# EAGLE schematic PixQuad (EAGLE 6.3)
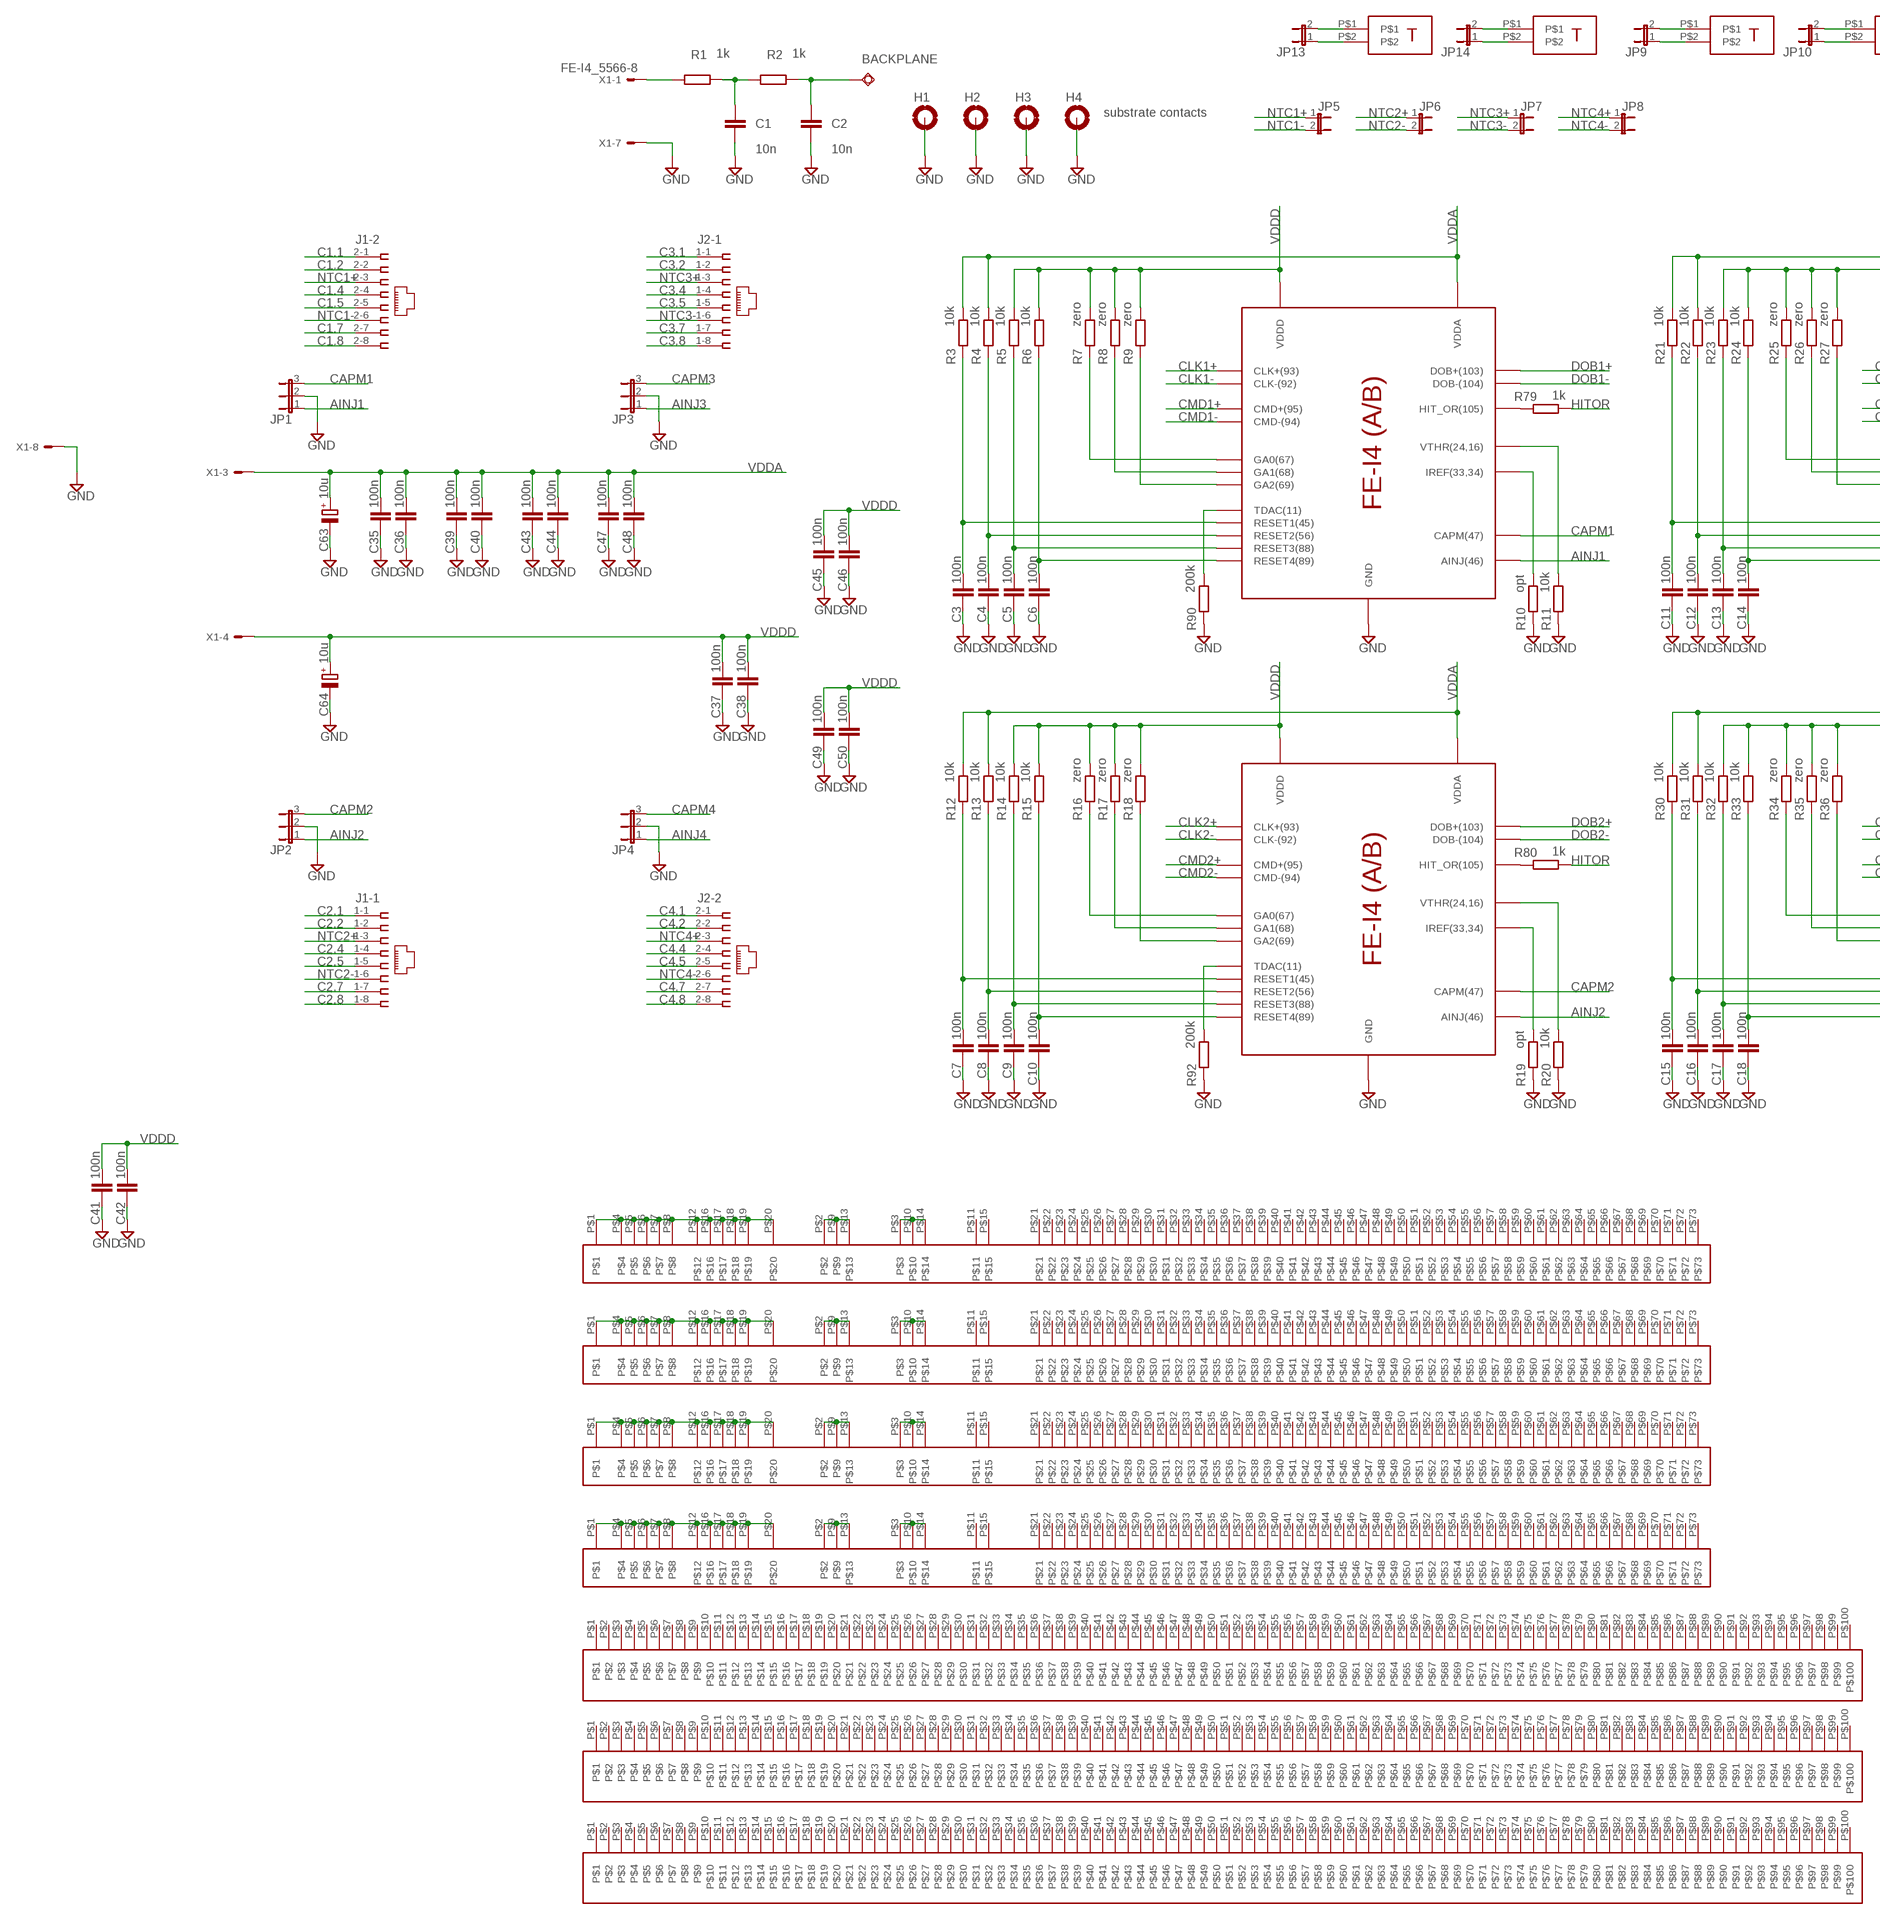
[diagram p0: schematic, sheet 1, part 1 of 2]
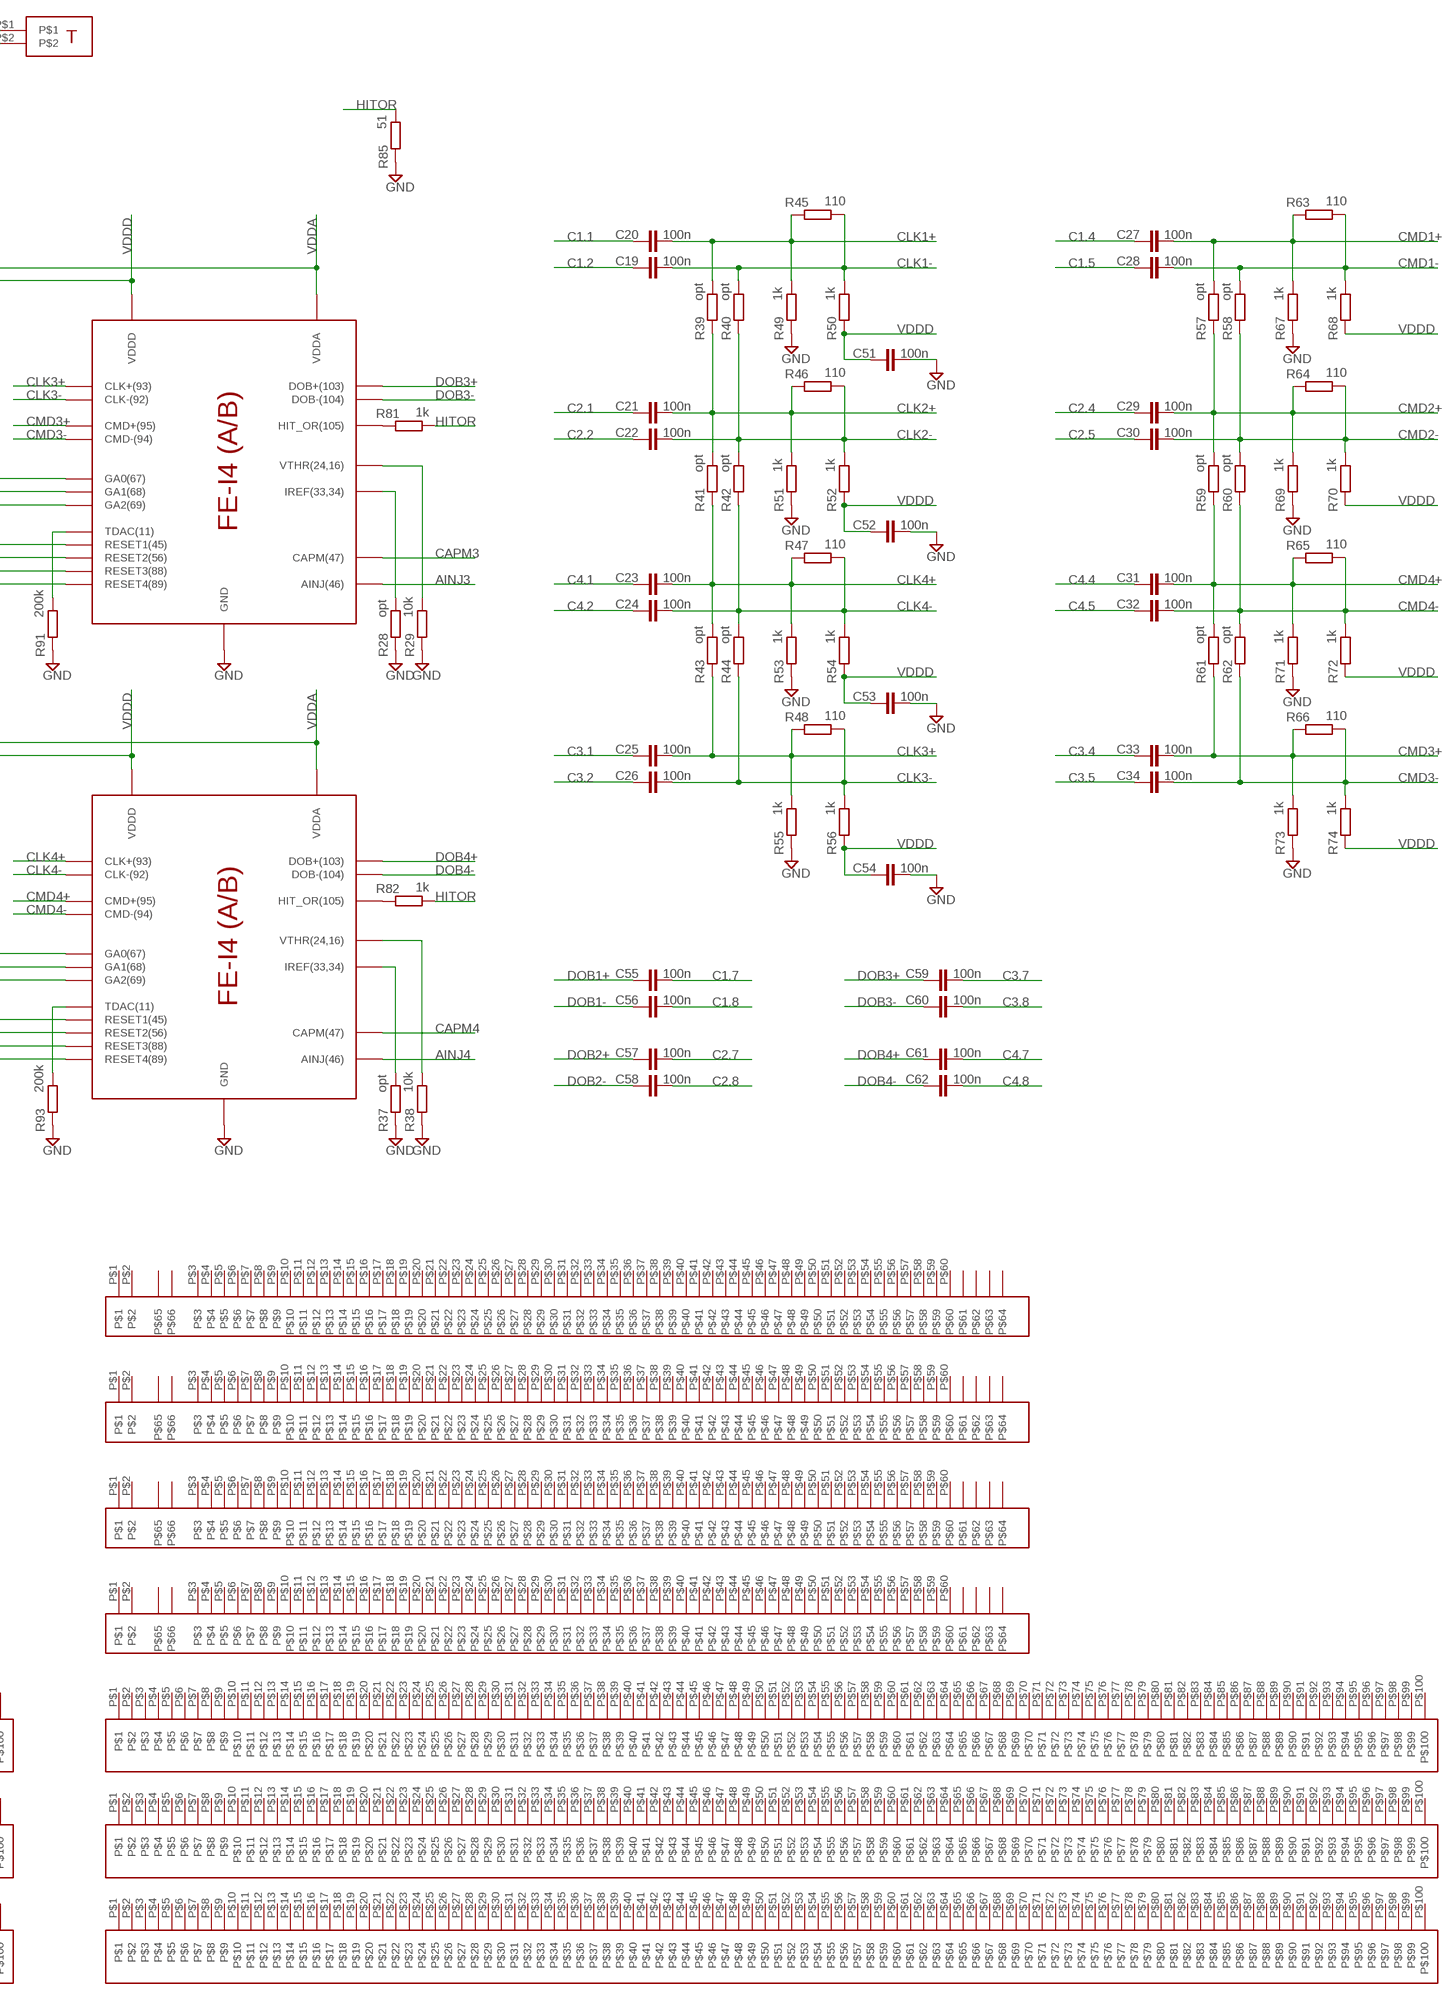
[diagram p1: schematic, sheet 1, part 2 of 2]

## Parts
BACKPLANE  TPSQTP20SQ  [TP20SQ]
C1  10n  C-EUC1210  [C1210]
C2  10n  C-EUC1210  [C1210]
C3  100n  C-EUC0402  [C0402]
C4  100n  C-EUC0402  [C0402]
C5  100n  C-EUC0402  [C0402]
C6  100n  C-EUC0402  [C0402]
C7  100n  C-EUC0402  [C0402]
C8  100n  C-EUC0402  [C0402]
C9  100n  C-EUC0402  [C0402]
C10  100n  C-EUC0402  [C0402]
C11  100n  C-EUC0402  [C0402]
C12  100n  C-EUC0402  [C0402]
C13  100n  C-EUC0402  [C0402]
C14  100n  C-EUC0402  [C0402]
C15  100n  C-EUC0402  [C0402]
C16  100n  C-EUC0402  [C0402]
C17  100n  C-EUC0402  [C0402]
C18  100n  C-EUC0402  [C0402]
C19  100n  C-EUC0402  [C0402]
C20  100n  C-EUC0402  [C0402]
C21  100n  C-EUC0402  [C0402]
C22  100n  C-EUC0402  [C0402]
C23  100n  C-EUC0402  [C0402]
C24  100n  C-EUC0402  [C0402]
C25  100n  C-EUC0402  [C0402]
C26  100n  C-EUC0402  [C0402]
C27  100n  C-EUC0402  [C0402]
C28  100n  C-EUC0402  [C0402]
C29  100n  C-EUC0402  [C0402]
C30  100n  C-EUC0402  [C0402]
C31  100n  C-EUC0402  [C0402]
C32  100n  C-EUC0402  [C0402]
C33  100n  C-EUC0402  [C0402]
C34  100n  C-EUC0402  [C0402]
C35  100n  C-EUC0402  [C0402]
C36  100n  C-EUC0402  [C0402]
C37  100n  C-EUC0402  [C0402]
C38  100n  C-EUC0402  [C0402]
C39  100n  C-EUC0402  [C0402]
C40  100n  C-EUC0402  [C0402]
C41  100n  C-EUC0402  [C0402]
C42  100n  C-EUC0402  [C0402]
C43  100n  C-EUC0402  [C0402]
C44  100n  C-EUC0402  [C0402]
C45  100n  C-EUC0402  [C0402]
C46  100n  C-EUC0402  [C0402]
C47  100n  C-EUC0402  [C0402]
C48  100n  C-EUC0402  [C0402]
C49  100n  C-EUC0402  [C0402]
C50  100n  C-EUC0402  [C0402]
C51  100n  C-EUC0402  [C0402]
C52  100n  C-EUC0402  [C0402]
C53  100n  C-EUC0402  [C0402]
C54  100n  C-EUC0402  [C0402]
C55  100n  C-EUC0402  [C0402]
C56  100n  C-EUC0402  [C0402]
C57  100n  C-EUC0402  [C0402]
C58  100n  C-EUC0402  [C0402]
C59  100n  C-EUC0402  [C0402]
C60  100n  C-EUC0402  [C0402]
C61  100n  C-EUC0402  [C0402]
C62  100n  C-EUC0402  [C0402]
C63  10u  CPOL-EUCT3528  [CT3528]
C64  10u  CPOL-EUCT3528  [CT3528]
H1  MOUNT-PAD-ROUND3.2  [3,2-PAD]
H2  MOUNT-PAD-ROUND3.2  [3,2-PAD]
H3  MOUNT-PAD-ROUND3.2  [3,2-PAD]
H4  substrate contacts  MOUNT-PAD-ROUND3.2  [3,2-PAD]
J1  557560-1  [557560-1]
J2  557560-1  [557560-1]
JP1  JP2E  [JP2]
JP2  JP2E  [JP2]
JP3  JP2E  [JP2]
JP4  JP2E  [JP2]
JP5  JP1E  [JP1]
JP6  JP1E  [JP1]
JP7  JP1E  [JP1]
JP8  JP1E  [JP1]
JP9  JP1E  [JUMPER_JP1]
JP10  JP1E  [JUMPER_JP1]
JP13  JP1E  [JUMPER_JP1]
JP14  JP1E  [JUMPER_JP1]
R1  1k  R-EU_R1206  [R1206]
R2  1k  R-EU_R1206  [R1206]
R3  10k  R-EU_R0402  [R0402]
R4  10k  R-EU_R0402  [R0402]
R5  10k  R-EU_R0402  [R0402]
R6  10k  R-EU_R0402  [R0402]
R7  zero  R-EU_R0402  [R0402]
R8  zero  R-EU_R0402  [R0402]
R9  zero  R-EU_R0402  [R0402]
R10  opt  R-EU_R0402  [R0402]
R11  10k  R-EU_R0402  [R0402]
R12  10k  R-EU_R0402  [R0402]
R13  10k  R-EU_R0402  [R0402]
R14  10k  R-EU_R0402  [R0402]
R15  10k  R-EU_R0402  [R0402]
R16  zero  R-EU_R0402  [R0402]
R17  zero  R-EU_R0402  [R0402]
R18  zero  R-EU_R0402  [R0402]
R19  opt  R-EU_R0402  [R0402]
R20  10k  R-EU_R0402  [R0402]
R21  10k  R-EU_R0402  [R0402]
R22  10k  R-EU_R0402  [R0402]
R23  10k  R-EU_R0402  [R0402]
R24  10k  R-EU_R0402  [R0402]
R25  zero  R-EU_R0402  [R0402]
R26  zero  R-EU_R0402  [R0402]
R27  zero  R-EU_R0402  [R0402]
R28  opt  R-EU_R0402  [R0402]
R29  10k  R-EU_R0402  [R0402]
R30  10k  R-EU_R0402  [R0402]
R31  10k  R-EU_R0402  [R0402]
R32  10k  R-EU_R0402  [R0402]
R33  10k  R-EU_R0402  [R0402]
R34  zero  R-EU_R0402  [R0402]
R35  zero  R-EU_R0402  [R0402]
R36  zero  R-EU_R0402  [R0402]
R37  opt  R-EU_R0402  [R0402]
R38  10k  R-EU_R0402  [R0402]
R39  opt  R-EU_R0402  [R0402]
R40  opt  R-EU_R0402  [R0402]
R41  opt  R-EU_R0402  [R0402]
R42  opt  R-EU_R0402  [R0402]
R43  opt  R-EU_R0402  [R0402]
R44  opt  R-EU_R0402  [R0402]
R45  110  R-EU_R0402  [R0402]
R46  110  R-EU_R0402  [R0402]
R47  110  R-EU_R0402  [R0402]
R48  110  R-EU_R0402  [R0402]
R49  1k  R-EU_R0402  [R0402]
R50  1k  R-EU_R0402  [R0402]
R51  1k  R-EU_R0402  [R0402]
R52  1k  R-EU_R0402  [R0402]
R53  1k  R-EU_R0402  [R0402]
R54  1k  R-EU_R0402  [R0402]
R55  1k  R-EU_R0402  [R0402]
R56  1k  R-EU_R0402  [R0402]
R57  opt  R-EU_R0402  [R0402]
R58  opt  R-EU_R0402  [R0402]
R59  opt  R-EU_R0402  [R0402]
R60  opt  R-EU_R0402  [R0402]
R61  opt  R-EU_R0402  [R0402]
R62  opt  R-EU_R0402  [R0402]
R63  110  R-EU_R0402  [R0402]
R64  110  R-EU_R0402  [R0402]
R65  110  R-EU_R0402  [R0402]
R66  110  R-EU_R0402  [R0402]
R67  1k  R-EU_R0402  [R0402]
R68  1k  R-EU_R0402  [R0402]
R69  1k  R-EU_R0402  [R0402]
R70  1k  R-EU_R0402  [R0402]
R71  1k  R-EU_R0402  [R0402]
R72  1k  R-EU_R0402  [R0402]
R73  1k  R-EU_R0402  [R0402]
R74  1k  R-EU_R0402  [R0402]
R79  1k  R-EU_R0402  [R0402]
R80  1k  R-EU_R0402  [R0402]
R81  1k  R-EU_R0402  [R0402]
R82  1k  R-EU_R0402  [R0402]
R85  51  RCL_R-EU_R0603  [RCL_R0603]
R90  200k  R-EU_R0402  [R0402]
R91  200k  R-EU_R0402  [R0402]
R92  200k  R-EU_R0402  [R0402]
R93  200k  R-EU_R0402  [R0402]
U$1  FE_I4ASIC  [FE-I4]
U$2  FE_I4ASIC  [FE-I4]
U$3  FE_I4ASIC  [FE-I4]
U$4  FE_I4ASIC  [FE-I4]
U$5  PA2  [PA2]
U$6  PA2  [PA2]
U$7  PA2  [PA2]
U$8  PA2  [PA2]
U$9  PA2  [PA2]
U$10  PA2  [PA2]
U$11  PA3  [PA3]
U$12  PA1  [PA1]
U$13  PA1  [PA1]
U$14  PA1  [PA1]
U$15  PA1  [PA1]
U$16  PA3  [PA3]
U$17  DORT  [DORT]
U$18  DORT  [DORT]
U$19  PA3  [PA3]
U$20  PA3  [PA3]
U$21  DORT  [DORT]
U$22  DORT  [DORT]
X1  FE-I4_5566-8  [FE-I4_5566-8]

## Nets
AINJ1: JP1.1 U$1.AINJ(46)
AINJ2: JP2.1 U$2.AINJ(46)
AINJ3: JP3.1 U$3.AINJ(46)
AINJ4: JP4.1 U$4.AINJ(46)
C1.1: C20.2 J1.2-1
C1.2: C19.2 J1.2-2
C1.4: C27.2 J1.2-4
C1.5: C28.2 J1.2-5
C1.7: C55.1 J1.2-7
C1.8: C56.1 J1.2-8
C2.1: C21.2 J1.1-1
C2.2: C22.2 J1.1-2
C2.4: C29.2 J1.1-4
C2.5: C30.2 J1.1-5
C2.7: C57.1 J1.1-7
C2.8: C58.1 J1.1-8
C3.1: C25.2 J2.1-1
C3.2: C26.2 J2.1-2
C3.4: C33.2 J2.1-4
C3.5: C34.2 J2.1-5
C3.7: C59.1 J2.1-7
C3.8: C60.1 J2.1-8
C4.1: C23.2 J2.2-1
C4.2: C24.2 J2.2-2
C4.4: C31.2 J2.2-4
C4.5: C32.2 J2.2-5
C4.7: C61.1 J2.2-7
C4.8: C62.1 J2.2-8
CAPM1: JP1.3 U$1.CAPM(47)
CAPM2: JP2.3 U$2.CAPM(47)
CAPM3: JP3.3 U$3.CAPM(47)
CAPM4: JP4.3 U$4.CAPM(47)
CLK1+: C20.1 R39.2 R45.1 R49.2 U$1.CLK+(93)
CLK1-: C19.1 R40.2 R45.2 R50.2 U$1.CLK-(92)
CLK2+: C21.1 R39.1 R41.2 R46.1 R51.2 U$2.CLK+(93)
CLK2-: C22.1 R40.1 R42.2 R46.2 R52.2 U$2.CLK-(92)
CLK3+: C25.1 R43.1 R48.1 R55.2 U$3.CLK+(93)
CLK3-: C26.1 R44.1 R48.2 R56.2 U$3.CLK-(92)
CLK4+: C23.1 R41.1 R43.2 R47.1 R53.2 U$4.CLK+(93)
CLK4-: C24.1 R42.1 R44.2 R47.2 R54.2 U$4.CLK-(92)
CMD1+: C27.1 R57.2 R63.1 R67.2 U$1.CMD+(95)
CMD1-: C28.1 R58.2 R63.2 R68.2 U$1.CMD-(94)
CMD2+: C29.1 R57.1 R59.2 R64.1 R69.2 U$2.CMD+(95)
CMD2-: C30.1 R58.1 R60.2 R64.2 R70.2 U$2.CMD-(94)
CMD3+: C33.1 R61.1 R66.1 R73.2 U$3.CMD+(95)
CMD3-: C34.1 R62.1 R66.2 R74.2 U$3.CMD-(94)
CMD4+: C31.1 R59.1 R61.2 R65.1 R71.2 U$4.CMD+(95)
CMD4-: C32.1 R60.1 R62.2 R65.2 R72.2 U$4.CMD-(94)
DOB1+: C55.2 U$1.DOB+(103)
DOB1-: C56.2 U$1.DOB-(104)
DOB2+: C57.2 U$2.DOB+(103)
DOB2-: C58.2 U$2.DOB-(104)
DOB3+: C59.2 U$3.DOB+(103)
DOB3-: C60.2 U$3.DOB-(104)
DOB4+: C61.2 U$4.DOB+(103)
DOB4-: C62.2 U$4.DOB-(104)
GND: C1.2 C2.2 C3.2 C4.2 C5.2 C6.2 C7.2 C8.2 C9.2 C10.2 C11.2 C12.2 C13.2 C14.2 C15.2 C16.2 C17.2 C18.2 C35.2 C36.2 C37.2 C38.2 C39.2 C40.2 C41.2 C42.2 C43.2 C44.2 C45.2 C46.2 C47.2 C48.2 C49.2 C50.2 C51.1 C52.1 C53.1 C54.1 C63.- C64.- H1.B3,2(MOUNT) H2.B3,2(MOUNT) H3.B3,2(MOUNT) H4.B3,2(MOUNT) JP1.2 JP2.2 JP3.2 JP4.2 R10.1 R11.1 R19.1 R20.1 R28.1 R29.1 R37.1 R38.1 R49.1 R51.1 R53.1 R55.1 R67.1 R69.1 R71.1 R73.1 R85.1 R90.1 R91.1 R92.1 R93.1 U$1.GND U$2.GND U$3.GND U$4.GND X1.7 X1.8
HITOR: R79.2 R80.2 R81.2 R82.2 R85.2
N$1: BACKPLANE.TP C2.1 R2.2
N$2: C1.1 R1.2 R2.1
N$3: JP13.2 U$17.P$1
N$4: C3.1 R3.1 U$1.RESET1(45)
N$5: C4.1 R4.1 U$1.RESET2(56)
N$6: C5.1 R5.1 U$1.RESET3(88)
N$7: C6.1 R6.1 U$1.RESET4(89)
N$8: R7.1 U$1.GA0(67)
N$9: R8.1 U$1.GA1(68)
N$10: R9.1 U$1.GA2(69)
N$11: R10.2 U$1.IREF(33,34)
N$12: R11.2 U$1.VTHR(24,16)
N$13: R79.1 U$1.P$1(HIT_OR(105))
N$14: R16.1 U$2.GA0(67)
N$15: R17.1 U$2.GA1(68)
N$16: R18.1 U$2.GA2(69)
N$17: C7.1 R12.1 U$2.RESET1(45)
N$18: C8.1 R13.1 U$2.RESET2(56)
N$19: C9.1 R14.1 U$2.RESET3(88)
N$20: C10.1 R15.1 U$2.RESET4(89)
N$21: R80.1 U$2.P$1(HIT_OR(105))
N$22: R81.1 U$3.P$1(HIT_OR(105))
N$23: R82.1 U$4.P$1(HIT_OR(105))
N$24: R90.2 U$1.TDAC(11)
N$25: R19.2 U$2.IREF(33,34)
N$26: R20.2 U$2.VTHR(24,16)
N$27: R91.2 U$3.TDAC(11)
N$28: R92.2 U$2.TDAC(11)
N$29: R93.2 U$4.TDAC(11)
N$30: JP13.1 U$17.P$2
N$31: JP14.1 U$18.P$2
N$32: JP14.2 U$18.P$1
N$33: U$11.P$1 U$11.P$4 U$11.P$5 U$11.P$6 U$11.P$7 U$11.P$8 U$11.P$12 U$11.P$16 U$11.P$17 U$11.P$18 U$11.P$19 U$11.P$20
N$34: R1.1 X1.1
N$35: U$16.P$1 U$16.P$4 U$16.P$5 U$16.P$6 U$16.P$7 U$16.P$8 U$16.P$12 U$16.P$16 U$16.P$17 U$16.P$18 U$16.P$19 U$16.P$20
N$36: U$19.P$1 U$19.P$4 U$19.P$5 U$19.P$6 U$19.P$7 U$19.P$8 U$19.P$12 U$19.P$16 U$19.P$17 U$19.P$18 U$19.P$19 U$19.P$20
N$37: U$20.P$1 U$20.P$4 U$20.P$5 U$20.P$6 U$20.P$7 U$20.P$8 U$20.P$12 U$20.P$16 U$20.P$17 U$20.P$18 U$20.P$19 U$20.P$20
N$38: U$11.P$2 U$11.P$9 U$11.P$13
N$39: U$16.P$2 U$16.P$9 U$16.P$13
N$40: U$19.P$2 U$19.P$9 U$19.P$13
N$41: U$20.P$2 U$20.P$9 U$20.P$13
N$42: U$20.P$3 U$20.P$10 U$20.P$14
N$43: U$19.P$3 U$19.P$10 U$19.P$14
N$44: U$16.P$3 U$16.P$10 U$16.P$14
N$45: U$11.P$3 U$11.P$10 U$11.P$14
N$46: JP9.1 U$21.P$2
N$47: JP9.2 U$21.P$1
N$48: JP10.1 U$22.P$2
N$49: JP10.2 U$22.P$1
N$50: R27.1 U$3.GA2(69)
N$56: R28.2 U$3.IREF(33,34)
N$57: R26.1 U$3.GA1(68)
N$58: R25.1 U$3.GA0(67)
N$59: C11.1 R21.1 U$3.RESET1(45)
N$60: C12.1 R22.1 U$3.RESET2(56)
N$61: C13.1 R23.1 U$3.RESET3(88)
N$62: C14.1 R24.1 U$3.RESET4(89)
N$64: R29.2 U$3.VTHR(24,16)
N$73: R34.1 U$4.GA0(67)
N$74: R35.1 U$4.GA1(68)
N$75: R36.1 U$4.GA2(69)
N$76: C15.1 R30.1 U$4.RESET1(45)
N$77: C16.1 R31.1 U$4.RESET2(56)
N$78: C17.1 R32.1 U$4.RESET3(88)
N$79: C18.1 R33.1 U$4.RESET4(89)
N$80: R37.2 U$4.IREF(33,34)
N$81: R38.2 U$4.VTHR(24,16)
NTC1+: J1.2-3 JP5.1
NTC1-: J1.2-6 JP5.2
NTC2+: J1.1-3 JP6.1
NTC2-: J1.1-6 JP6.2
NTC3+: J2.1-3 JP7.1
NTC3-: J2.1-6 JP7.2
NTC4+: J2.2-3 JP8.1
NTC4-: J2.2-6 JP8.2
VDDA: C35.1 C36.1 C39.1 C40.1 C43.1 C44.1 C47.1 C48.1 C63.+ R3.2 R4.2 R12.2 R13.2 R21.2 R22.2 R30.2 R31.2 U$1.VDDA U$2.VDDA U$3.VDDA U$4.VDDA X1.3
VDDD: C37.1 C38.1 C41.1 C42.1 C45.1 C46.1 C49.1 C50.1 C51.2 C52.2 C53.2 C54.2 C64.+ R5.2 R6.2 R7.2 R8.2 R9.2 R14.2 R15.2 R16.2 R17.2 R18.2 R23.2 R24.2 R25.2 R26.2 R27.2 R32.2 R33.2 R34.2 R35.2 R36.2 R50.1 R52.1 R54.1 R56.1 R68.1 R70.1 R72.1 R74.1 U$1.VDDD U$2.VDDD U$3.VDDD U$4.VDDD X1.4
Unconnected: U$5.P$1 U$5.P$2 U$5.P$3 U$5.P$4 U$5.P$5 U$5.P$6 U$5.P$7 U$5.P$8 U$5.P$9 U$5.P$10 U$5.P$11 U$5.P$12 U$5.P$13 U$5.P$14 U$5.P$15 U$5.P$16 U$5.P$17 U$5.P$18 U$5.P$19 U$5.P$20 U$5.P$21 U$5.P$22 U$5.P$23 U$5.P$24 U$5.P$25 U$5.P$26 U$5.P$27 U$5.P$28 U$5.P$29 U$5.P$30 U$5.P$31 U$5.P$32 U$5.P$33 U$5.P$34 U$5.P$35 U$5.P$36 U$5.P$37 U$5.P$38 U$5.P$39 U$5.P$40 U$5.P$41 U$5.P$42 U$5.P$43 U$5.P$44 U$5.P$45 U$5.P$46 U$5.P$47 U$5.P$48 U$5.P$49 U$5.P$50 U$5.P$51 U$5.P$52 U$5.P$53 U$5.P$54 U$5.P$55 U$5.P$56 U$5.P$57 U$5.P$58 U$5.P$59 U$5.P$60 U$5.P$61 U$5.P$62 U$5.P$63 U$5.P$64 U$5.P$65 U$5.P$66 U$5.P$67 U$5.P$68 U$5.P$69 U$5.P$70 U$5.P$71 U$5.P$72 U$5.P$73 U$5.P$74 U$5.P$75 U$5.P$76 U$5.P$77 U$5.P$78 U$5.P$79 U$5.P$80 U$5.P$81 U$5.P$82 U$5.P$83 U$5.P$84 U$5.P$85 U$5.P$86 U$5.P$87 U$5.P$88 U$5.P$89 U$5.P$90 U$5.P$91 U$5.P$92 U$5.P$93 U$5.P$94 U$5.P$95 U$5.P$96 U$5.P$97 U$5.P$98 U$5.P$99 U$5.P$100 U$6.P$1 U$6.P$2 U$6.P$3 U$6.P$4 U$6.P$5 U$6.P$6 U$6.P$7 U$6.P$8 U$6.P$9 U$6.P$10 U$6.P$11 U$6.P$12 U$6.P$13 U$6.P$14 U$6.P$15 U$6.P$16 U$6.P$17 U$6.P$18 U$6.P$19 U$6.P$20 U$6.P$21 U$6.P$22 U$6.P$23 U$6.P$24 U$6.P$25 U$6.P$26 U$6.P$27 U$6.P$28 U$6.P$29 U$6.P$30 U$6.P$31 U$6.P$32 U$6.P$33 U$6.P$34 U$6.P$35 U$6.P$36 U$6.P$37 U$6.P$38 U$6.P$39 U$6.P$40 U$6.P$41 U$6.P$42 U$6.P$43 U$6.P$44 U$6.P$45 U$6.P$46 U$6.P$47 U$6.P$48 U$6.P$49 U$6.P$50 U$6.P$51 U$6.P$52 U$6.P$53 U$6.P$54 U$6.P$55 U$6.P$56 U$6.P$57 U$6.P$58 U$6.P$59 U$6.P$60 U$6.P$61 U$6.P$62 U$6.P$63 U$6.P$64 U$6.P$65 U$6.P$66 U$6.P$67 U$6.P$68 U$6.P$69 U$6.P$70 U$6.P$71 U$6.P$72 U$6.P$73 U$6.P$74 U$6.P$75 U$6.P$76 U$6.P$77 U$6.P$78 U$6.P$79 U$6.P$80 U$6.P$81 U$6.P$82 U$6.P$83 U$6.P$84 U$6.P$85 U$6.P$86 U$6.P$87 U$6.P$88 U$6.P$89 U$6.P$90 U$6.P$91 U$6.P$92 U$6.P$93 U$6.P$94 U$6.P$95 U$6.P$96 U$6.P$97 U$6.P$98 U$6.P$99 U$6.P$100 U$7.P$1 U$7.P$2 U$7.P$3 U$7.P$4 U$7.P$5 U$7.P$6 U$7.P$7 U$7.P$8 U$7.P$9 U$7.P$10 U$7.P$11 U$7.P$12 U$7.P$13 U$7.P$14 U$7.P$15 U$7.P$16 U$7.P$17 U$7.P$18 U$7.P$19 U$7.P$20 U$7.P$21 U$7.P$22 U$7.P$23 U$7.P$24 U$7.P$25 U$7.P$26 U$7.P$27 U$7.P$28 U$7.P$29 U$7.P$30 U$7.P$31 U$7.P$32 U$7.P$33 U$7.P$34 U$7.P$35 U$7.P$36 U$7.P$37 U$7.P$38 U$7.P$39 U$7.P$40 U$7.P$41 U$7.P$42 U$7.P$43 U$7.P$44 U$7.P$45 U$7.P$46 U$7.P$47 U$7.P$48 U$7.P$49 U$7.P$50 U$7.P$51 U$7.P$52 U$7.P$53 U$7.P$54 U$7.P$55 U$7.P$56 U$7.P$57 U$7.P$58 U$7.P$59 U$7.P$60 U$7.P$61 U$7.P$62 U$7.P$63 U$7.P$64 U$7.P$65 U$7.P$66 U$7.P$67 U$7.P$68 U$7.P$69 U$7.P$70 U$7.P$71 U$7.P$72 U$7.P$73 U$7.P$74 U$7.P$75 U$7.P$76 U$7.P$77 U$7.P$78 U$7.P$79 U$7.P$80 U$7.P$81 U$7.P$82 U$7.P$83 U$7.P$84 U$7.P$85 U$7.P$86 U$7.P$87 U$7.P$88 U$7.P$89 U$7.P$90 U$7.P$91 U$7.P$92 U$7.P$93 U$7.P$94 U$7.P$95 U$7.P$96 U$7.P$97 U$7.P$98 U$7.P$99 U$7.P$100 U$8.P$1 U$8.P$2 U$8.P$3 U$8.P$4 U$8.P$5 U$8.P$6 U$8.P$7 U$8.P$8 U$8.P$9 U$8.P$10 U$8.P$11 U$8.P$12 U$8.P$13 U$8.P$14 U$8.P$15 U$8.P$16 U$8.P$17 U$8.P$18 U$8.P$19 U$8.P$20 U$8.P$21 U$8.P$22 U$8.P$23 U$8.P$24 U$8.P$25 U$8.P$26 U$8.P$27 U$8.P$28 U$8.P$29 U$8.P$30 U$8.P$31 U$8.P$32 U$8.P$33 U$8.P$34 U$8.P$35 U$8.P$36 U$8.P$37 U$8.P$38 U$8.P$39 U$8.P$40 U$8.P$41 U$8.P$42 U$8.P$43 U$8.P$44 U$8.P$45 U$8.P$46 U$8.P$47 U$8.P$48 U$8.P$49 U$8.P$50 U$8.P$51 U$8.P$52 U$8.P$53 U$8.P$54 U$8.P$55 U$8.P$56 U$8.P$57 U$8.P$58 U$8.P$59 U$8.P$60 U$8.P$61 U$8.P$62 U$8.P$63 U$8.P$64 U$8.P$65 U$8.P$66 U$8.P$67 U$8.P$68 U$8.P$69 U$8.P$70 U$8.P$71 U$8.P$72 U$8.P$73 U$8.P$74 U$8.P$75 U$8.P$76 U$8.P$77 U$8.P$78 U$8.P$79 U$8.P$80 U$8.P$81 U$8.P$82 U$8.P$83 U$8.P$84 U$8.P$85 U$8.P$86 U$8.P$87 U$8.P$88 U$8.P$89 U$8.P$90 U$8.P$91 U$8.P$92 U$8.P$93 U$8.P$94 U$8.P$95 U$8.P$96 U$8.P$97 U$8.P$98 U$8.P$99 U$8.P$100 U$9.P$1 U$9.P$2 U$9.P$3 U$9.P$4 U$9.P$5 U$9.P$6 U$9.P$7 U$9.P$8 U$9.P$9 U$9.P$10 U$9.P$11 U$9.P$12 U$9.P$13 U$9.P$14 U$9.P$15 U$9.P$16 U$9.P$17 U$9.P$18 U$9.P$19 U$9.P$20 U$9.P$21 U$9.P$22 U$9.P$23 U$9.P$24 U$9.P$25 U$9.P$26 U$9.P$27 U$9.P$28 U$9.P$29 U$9.P$30 U$9.P$31 U$9.P$32 U$9.P$33 U$9.P$34 U$9.P$35 U$9.P$36 U$9.P$37 U$9.P$38 U$9.P$39 U$9.P$40 U$9.P$41 U$9.P$42 U$9.P$43 U$9.P$44 U$9.P$45 U$9.P$46 U$9.P$47 U$9.P$48 U$9.P$49 U$9.P$50 U$9.P$51 U$9.P$52 U$9.P$53 U$9.P$54 U$9.P$55 U$9.P$56 U$9.P$57 U$9.P$58 U$9.P$59 U$9.P$60 U$9.P$61 U$9.P$62 U$9.P$63 U$9.P$64 U$9.P$65 U$9.P$66 U$9.P$67 U$9.P$68 U$9.P$69 U$9.P$70 U$9.P$71 U$9.P$72 U$9.P$73 U$9.P$74 U$9.P$75 U$9.P$76 U$9.P$77 U$9.P$78 U$9.P$79 U$9.P$80 U$9.P$81 U$9.P$82 U$9.P$83 U$9.P$84 U$9.P$85 U$9.P$86 U$9.P$87 U$9.P$88 U$9.P$89 U$9.P$90 U$9.P$91 U$9.P$92 U$9.P$93 U$9.P$94 U$9.P$95 U$9.P$96 U$9.P$97 U$9.P$98 U$9.P$99 U$9.P$100 U$10.P$1 U$10.P$2 U$10.P$3 U$10.P$4 U$10.P$5 U$10.P$6 U$10.P$7 U$10.P$8 U$10.P$9 U$10.P$10 U$10.P$11 U$10.P$12 U$10.P$13 U$10.P$14 U$10.P$15 U$10.P$16 U$10.P$17 U$10.P$18 U$10.P$19 U$10.P$20 U$10.P$21 U$10.P$22 U$10.P$23 U$10.P$24 U$10.P$25 U$10.P$26 U$10.P$27 U$10.P$28 U$10.P$29 U$10.P$30 U$10.P$31 U$10.P$32 U$10.P$33 U$10.P$34 U$10.P$35 U$10.P$36 U$10.P$37 U$10.P$38 U$10.P$39 U$10.P$40 U$10.P$41 U$10.P$42 U$10.P$43 U$10.P$44 U$10.P$45 U$10.P$46 U$10.P$47 U$10.P$48 U$10.P$49 U$10.P$50 U$10.P$51 U$10.P$52 U$10.P$53 U$10.P$54 U$10.P$55 U$10.P$56 U$10.P$57 U$10.P$58 U$10.P$59 U$10.P$60 U$10.P$61 U$10.P$62 U$10.P$63 U$10.P$64 U$10.P$65 U$10.P$66 U$10.P$67 U$10.P$68 U$10.P$69 U$10.P$70 U$10.P$71 U$10.P$72 U$10.P$73 U$10.P$74 U$10.P$75 U$10.P$76 U$10.P$77 U$10.P$78 U$10.P$79 U$10.P$80 U$10.P$81 U$10.P$82 U$10.P$83 U$10.P$84 U$10.P$85 U$10.P$86 U$10.P$87 U$10.P$88 U$10.P$89 U$10.P$90 U$10.P$91 U$10.P$92 U$10.P$93 U$10.P$94 U$10.P$95 U$10.P$96 U$10.P$97 U$10.P$98 U$10.P$99 U$10.P$100 U$11.P$11 U$11.P$15 U$11.P$21 U$11.P$22 U$11.P$23 U$11.P$24 U$11.P$25 U$11.P$26 U$11.P$27 U$11.P$28 U$11.P$29 U$11.P$30 U$11.P$31 U$11.P$32 U$11.P$33 U$11.P$34 U$11.P$35 U$11.P$36 U$11.P$37 U$11.P$38 U$11.P$39 U$11.P$40 U$11.P$41 U$11.P$42 U$11.P$43 U$11.P$44 U$11.P$45 U$11.P$46 U$11.P$47 U$11.P$48 U$11.P$49 U$11.P$50 U$11.P$51 U$11.P$52 U$11.P$53 U$11.P$54 U$11.P$55 U$11.P$56 U$11.P$57 U$11.P$58 U$11.P$59 U$11.P$60 U$11.P$61 U$11.P$62 U$11.P$63 U$11.P$64 U$11.P$65 U$11.P$66 U$11.P$67 U$11.P$68 U$11.P$69 U$11.P$70 U$11.P$71 U$11.P$72 U$11.P$73 U$12.P$1 U$12.P$2 U$12.P$3 U$12.P$4 U$12.P$5 U$12.P$6 U$12.P$7 U$12.P$8 U$12.P$9 U$12.P$10 U$12.P$11 U$12.P$12 U$12.P$13 U$12.P$14 U$12.P$15 U$12.P$16 U$12.P$17 U$12.P$18 U$12.P$19 U$12.P$20 U$12.P$21 U$12.P$22 U$12.P$23 U$12.P$24 U$12.P$25 U$12.P$26 U$12.P$27 U$12.P$28 U$12.P$29 U$12.P$30 U$12.P$31 U$12.P$32 U$12.P$33 U$12.P$34 U$12.P$35 U$12.P$36 U$12.P$37 U$12.P$38 U$12.P$39 U$12.P$40 U$12.P$41 U$12.P$42 U$12.P$43 U$12.P$44 U$12.P$45 U$12.P$46 U$12.P$47 U$12.P$48 U$12.P$49 U$12.P$50 U$12.P$51 U$12.P$52 U$12.P$53 U$12.P$54 U$12.P$55 U$12.P$56 U$12.P$57 U$12.P$58 U$12.P$59 U$12.P$60 U$12.P$61 U$12.P$62 U$12.P$63 U$12.P$64 U$12.P$65 U$12.P$66 U$13.P$1 U$13.P$2 U$13.P$3 U$13.P$4 U$13.P$5 U$13.P$6 U$13.P$7 U$13.P$8 U$13.P$9 U$13.P$10 U$13.P$11 U$13.P$12 U$13.P$13 U$13.P$14 U$13.P$15 U$13.P$16 U$13.P$17 U$13.P$18 U$13.P$19 U$13.P$20 U$13.P$21 U$13.P$22 U$13.P$23 U$13.P$24 U$13.P$25 U$13.P$26 U$13.P$27 U$13.P$28 U$13.P$29 U$13.P$30 U$13.P$31 U$13.P$32 U$13.P$33 U$13.P$34 U$13.P$35 U$13.P$36 U$13.P$37 U$13.P$38 U$13.P$39 U$13.P$40 U$13.P$41 U$13.P$42 U$13.P$43 U$13.P$44 U$13.P$45 U$13.P$46 U$13.P$47 U$13.P$48 U$13.P$49 U$13.P$50 U$13.P$51 U$13.P$52 U$13.P$53 U$13.P$54 U$13.P$55 U$13.P$56 U$13.P$57 U$13.P$58 U$13.P$59 U$13.P$60 U$13.P$61 U$13.P$62 U$13.P$63 U$13.P$64 U$13.P$65 U$13.P$66 U$14.P$1 U$14.P$2 U$14.P$3 U$14.P$4 U$14.P$5 U$14.P$6 U$14.P$7 U$14.P$8 U$14.P$9 U$14.P$10 U$14.P$11 U$14.P$12 U$14.P$13 U$14.P$14 U$14.P$15 U$14.P$16 U$14.P$17 U$14.P$18 U$14.P$19 U$14.P$20 U$14.P$21 U$14.P$22 U$14.P$23 U$14.P$24 U$14.P$25 U$14.P$26 U$14.P$27 U$14.P$28 U$14.P$29 U$14.P$30 U$14.P$31 U$14.P$32 U$14.P$33 U$14.P$34 U$14.P$35 U$14.P$36 U$14.P$37 U$14.P$38 U$14.P$39 U$14.P$40 U$14.P$41 U$14.P$42 U$14.P$43 U$14.P$44 U$14.P$45 U$14.P$46 U$14.P$47 U$14.P$48 U$14.P$49 U$14.P$50 U$14.P$51 U$14.P$52 U$14.P$53 U$14.P$54 U$14.P$55 U$14.P$56 U$14.P$57 U$14.P$58 U$14.P$59 U$14.P$60 U$14.P$61 U$14.P$62 U$14.P$63 U$14.P$64 U$14.P$65 U$14.P$66 U$15.P$1 U$15.P$2 U$15.P$3 U$15.P$4 U$15.P$5 U$15.P$6 U$15.P$7 U$15.P$8 U$15.P$9 U$15.P$10 U$15.P$11 U$15.P$12 U$15.P$13 U$15.P$14 U$15.P$15 U$15.P$16 U$15.P$17 U$15.P$18 U$15.P$19 U$15.P$20 U$15.P$21 U$15.P$22 U$15.P$23 U$15.P$24 U$15.P$25 U$15.P$26 U$15.P$27 U$15.P$28 U$15.P$29 U$15.P$30 U$15.P$31 U$15.P$32 U$15.P$33 U$15.P$34 U$15.P$35 U$15.P$36 U$15.P$37 U$15.P$38 U$15.P$39 U$15.P$40 U$15.P$41 U$15.P$42 U$15.P$43 U$15.P$44 U$15.P$45 U$15.P$46 U$15.P$47 U$15.P$48 U$15.P$49 U$15.P$50 U$15.P$51 U$15.P$52 U$15.P$53 U$15.P$54 U$15.P$55 U$15.P$56 U$15.P$57 U$15.P$58 U$15.P$59 U$15.P$60 U$15.P$61 U$15.P$62 U$15.P$63 U$15.P$64 U$15.P$65 U$15.P$66 U$16.P$11 U$16.P$15 U$16.P$21 U$16.P$22 U$16.P$23 U$16.P$24 U$16.P$25 U$16.P$26 U$16.P$27 U$16.P$28 U$16.P$29 U$16.P$30 U$16.P$31 U$16.P$32 U$16.P$33 U$16.P$34 U$16.P$35 U$16.P$36 U$16.P$37 U$16.P$38 U$16.P$39 U$16.P$40 U$16.P$41 U$16.P$42 U$16.P$43 U$16.P$44 U$16.P$45 U$16.P$46 U$16.P$47 U$16.P$48 U$16.P$49 U$16.P$50 U$16.P$51 U$16.P$52 U$16.P$53 U$16.P$54 U$16.P$55 U$16.P$56 U$16.P$57 U$16.P$58 U$16.P$59 U$16.P$60 U$16.P$61 U$16.P$62 U$16.P$63 U$16.P$64 U$16.P$65 U$16.P$66 U$16.P$67 U$16.P$68 U$16.P$69 U$16.P$70 U$16.P$71 U$16.P$72 U$16.P$73 U$19.P$11 U$19.P$15 U$19.P$21 U$19.P$22 U$19.P$23 U$19.P$24 U$19.P$25 U$19.P$26 U$19.P$27 U$19.P$28 U$19.P$29 U$19.P$30 U$19.P$31 U$19.P$32 U$19.P$33 U$19.P$34 U$19.P$35 U$19.P$36 U$19.P$37 U$19.P$38 U$19.P$39 U$19.P$40 U$19.P$41 U$19.P$42 U$19.P$43 U$19.P$44 U$19.P$45 U$19.P$46 U$19.P$47 U$19.P$48 U$19.P$49 U$19.P$50 U$19.P$51 U$19.P$52 U$19.P$53 U$19.P$54 U$19.P$55 U$19.P$56 U$19.P$57 U$19.P$58 U$19.P$59 U$19.P$60 U$19.P$61 U$19.P$62 U$19.P$63 U$19.P$64 U$19.P$65 U$19.P$66 U$19.P$67 U$19.P$68 U$19.P$69 U$19.P$70 U$19.P$71 U$19.P$72 U$19.P$73 U$20.P$11 U$20.P$15 U$20.P$21 U$20.P$22 U$20.P$23 U$20.P$24 U$20.P$25 U$20.P$26 U$20.P$27 U$20.P$28 U$20.P$29 U$20.P$30 U$20.P$31 U$20.P$32 U$20.P$33 U$20.P$34 U$20.P$35 U$20.P$36 U$20.P$37 U$20.P$38 U$20.P$39 U$20.P$40 U$20.P$41 U$20.P$42 U$20.P$43 U$20.P$44 U$20.P$45 U$20.P$46 U$20.P$47 U$20.P$48 U$20.P$49 U$20.P$50 U$20.P$51 U$20.P$52 U$20.P$53 U$20.P$54 U$20.P$55 U$20.P$56 U$20.P$57 U$20.P$58 U$20.P$59 U$20.P$60 U$20.P$61 U$20.P$62 U$20.P$63 U$20.P$64 U$20.P$65 U$20.P$66 U$20.P$67 U$20.P$68 U$20.P$69 U$20.P$70 U$20.P$71 U$20.P$72 U$20.P$73

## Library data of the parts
BACKPLANE = testpad:TPSQ: Test pad
C1-C62 = rcl:C-EU: CAPACITOR, European symbol
C63 C64 = rcl:CPOL-EU: POLARIZED CAPACITOR, European symbol
H1-H4 = holes:MOUNT-PAD-ROUND: MOUNTING PAD, round
J1 J2 = con-amp:557560-1: AMP connector
JP1-JP4 = jumper:JP2E: JUMPER
JP5-JP8 = jumper:JP1E: JUMPER
JP9 JP10 JP13 JP14 = FE-I4:JP1E: JUMPER
R1-R74 R79-R82 R90-R93 = rcl:R-EU_: RESISTOR, European symbol
R85 = FE-I4:RCL_R-EU_: RESISTOR, European symbol
U$1-U$4 = FE-I4:FE_I4
U$5-U$10 = FE-I4:PA2
U$11 U$16 U$19 U$20 = FE-I4:PA3
U$12-U$15 = FE-I4:PA1
U$17 U$18 U$21 U$22 = FE-I4:DORT
X1 = FE-I4:FE-I4_5566-8: Mini FIT connector 8 pol Source: http://www.molex.com; OC_FARNELL: unknown; OC_NEWARK: unknown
